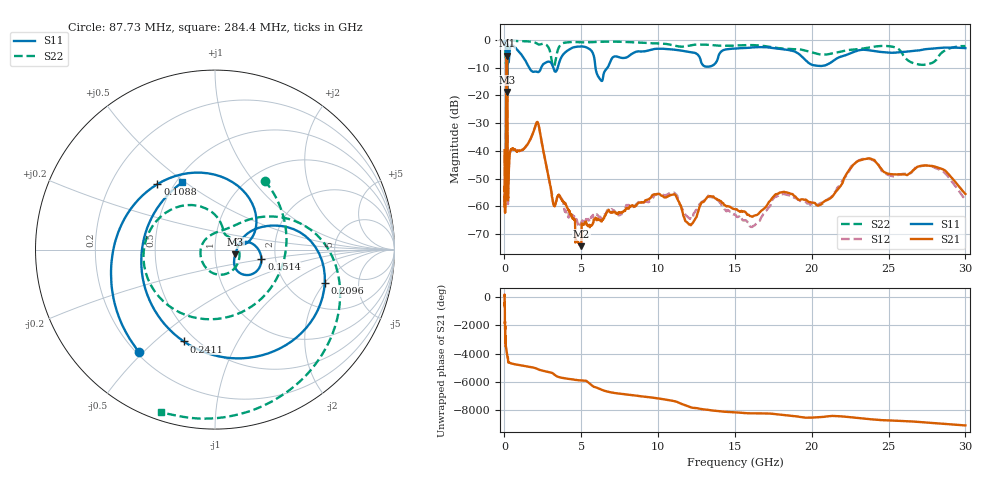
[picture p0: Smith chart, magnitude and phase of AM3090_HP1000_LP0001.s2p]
! Date/Time: Thu, Feb 28, 2019 2:01 PM
! Network Analyzer: Agilent Technologies E8364B Rev: A.07.50.67
! Sweep from 0.010 to 30.000 GHz, 1601 Points, Sweep Type: LOG
! Power Supply: 5.023 V, 0.002 A
# Hz S DB R 50
!freq MagS11 AngS11 MagS21 AngS21 MagS12 AngS12 MagS22 AngS22
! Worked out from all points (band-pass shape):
!   1601 points, 10 MHz to 30 GHz, reference 50 ohm
!   highest |S21| = -5.61 dB at 144.7 MHz (marker M1); lowest = -74.4 dB at 5.002 GHz (marker M2)
!   |S21| within 3 dB of the highest: 121 MHz to 180.5 MHz (59.49 MHz wide, 39.5 % of centre)
!   lowest |S11| = -18.7 dB at 180.3 MHz (marker M3), VSWR 1.26, Z = 62.6 - j3.4 ohm
!   |S11| at or under -10 dB: 1.609 GHz to 2.388 GHz (778.4 MHz wide, 39 % of centre); 3.182 GHz to 3.465 GHz (283.4 MHz wide, 8.53 % of centre); 5.926 GHz to 6.698 GHz (772.2 MHz wide, 12.2 % of centre)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
!   |S22| runs from -22.3 to -0.1 dB; largest |S21 - S12| = 0.018
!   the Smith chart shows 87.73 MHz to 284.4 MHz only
!   S11 on the Smith chart (normalised r, x): 87.73 MHz: 0.21, -0.48; 108.8 MHz: 0.41, +0.39; 151.4 MHz: 1.68, -0.18; 209.6 MHz: 3.19, -2.01; 241.1 MHz: 0.43, -0.62; 284.4 MHz: 0.54, +0.49
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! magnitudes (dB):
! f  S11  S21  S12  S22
! 10 MHz  -0.2  -39.8  -41.4  -0.5
! 38.04 MHz  -0.5  -61.6  -60.5  -1.3
! 48.61 MHz  -0.8  -48.6  -49.0  -1.5
! 87.73 MHz  -3.0  -50.1  -48.8  -6.5
! 108.8 MHz  -6.3  -19.8  -19.8  -7.8
! 144.7 MHz  -12.7  -5.6  -5.6  -17.4
! 151.4 MHz  -11.6  -5.7  -5.6  -16.5
! 180.3 MHz  -18.7  -8.6  -8.5  -19.3
! 209.6 MHz  -3.9  -48.6  -48.1  -2.5
! 241.1 MHz  -5.3  -55.4  -56.4  -0.7
! 284.4 MHz  -7.6  -47.2  -47.1  -0.4
! 550.5 MHz  -2.1  -39.3  -39.4  -0.2
! 2.084 GHz  -11.4  -29.9  -29.9  -1.2
! 3.22 GHz  -10.7  -59.7  -59.2  -9.6
! 5.002 GHz  -2.3  -74.4  -66.0  -0.8
! 6.202 GHz  -14.0  -64.9  -63.9  -0.6
! 7.926 GHz  -6.3  -60.7  -59.6  -0.7
! 10.81 GHz  -3.3  -55.9  -55.3  -1.7
! 16.13 GHz  -2.7  -63.8  -67.5  -1.8
! 20.72 GHz  -9.3  -58.7  -59.2  -5.2
! 23.48 GHz  -3.5  -43.0  -42.9  -2.9
! 30 GHz  -2.9  -55.6  -57.7  -2.2
